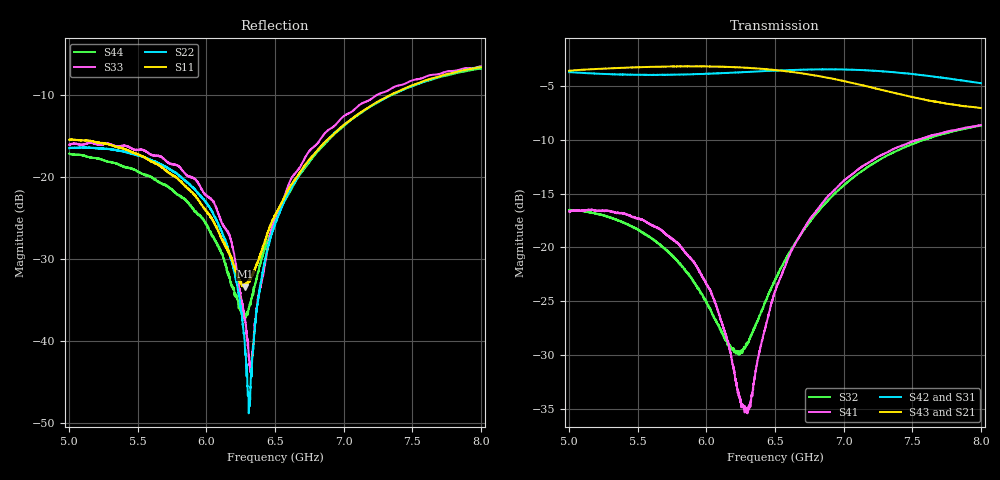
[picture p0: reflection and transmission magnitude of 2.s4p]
!Keysight Technologies,N5225A,MY51451420,A.10.40.12
!Date: Wednesday, May 11, 2016 10:17:49
!Correction: S11(Full 4 Port(1,2,3,4))
!S12(Full 4 Port(1,2,3,4))
!S13(Full 4 Port(1,2,3,4))
!S14(Full 4 Port(1,2,3,4))
!S21(Full 4 Port(1,2,3,4))
!S22(Full 4 Port(1,2,3,4))
!S23(Full 4 Port(1,2,3,4))
!S24(Full 4 Port(1,2,3,4))
!S31(Full 4 Port(1,2,3,4))
!S32(Full 4 Port(1,2,3,4))
!S33(Full 4 Port(1,2,3,4))
!S34(Full 4 Port(1,2,3,4))
!S41(Full 4 Port(1,2,3,4))
!S42(Full 4 Port(1,2,3,4))
!S43(Full 4 Port(1,2,3,4))
!S44(Full 4 Port(1,2,3,4))
!S4P File: Measurements: <S11,S12,S13,S14>,
!<S21,S22,S23,S24>,
!<S31,S32,S33,S34>,
!<S41,S42,S43,S44>:
# Hz S  dB  R 50
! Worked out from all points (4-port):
!   3201 points, 5 GHz to 8 GHz, reference 50 ohm
!   strongest paths, dB at 5 GHz, 5.75 GHz, 6.5 GHz, 7.25 GHz, 8 GHz:
!     S43: -3.6, -3.2, -3.5, -5.3, -7.0
!     S21: -3.6, -3.2, -3.5, -5.2, -7.1
!     S42: -3.7, -3.9, -3.6, -3.6, -4.7
!     S31: -3.8, -4.0, -3.6, -3.7, -4.8
!     S41: -16.7, -19.2, -24.1, -11.6, -8.6
!     S32: -16.5, -20.7, -23.0, -11.9, -8.7
!   lowest |S11| = -33.4 dB at 6.283 GHz (marker M1), VSWR 1.04, Z = 50.8 + j2.02 ohm
!   |S11| at or under -10 dB: start of sweep to 7.336 GHz
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5e9  -15.44 12.8  -3.62 104.7  -3.78 9.8  -16.65 171.5
     -3.62 104.7  -16.47 -113.1  -16.51 -78.1  -3.70 128.3
     -3.77 9.8  -16.50 -78.1  -16.06 -133.0  -3.56 -143.9
     -16.66 171.5  -3.71 128.3  -3.57 -143.9  -17.14 -121.3
5.691875e9  -18.99 -107.9  -3.22 7.5  -4.01 -86.6  -18.60 84.8
            -3.22 7.4  -18.66 162.0  -20.10 -142.1  -3.96 47.9
            -4.01 -86.6  -20.06 -142.0  -17.83 145.0  -3.19 134.1
            -18.61 84.8  -3.95 47.9  -3.19 134.1  -20.94 149.3
6.11e9  -27.42 158.3  -3.22 -52.0  -3.82 -145.9  -26.93 37.7
        -3.23 -52.0  -26.59 106.4  -27.87 -155.0  -3.81 -1.4
        -3.83 -146.0  -27.85 -155.0  -25.53 102.0  -3.21 84.0
        -26.89 37.6  -3.80 -1.5  -3.20 84.0  -29.22 84.7
6.283438e9  -33.37 67.8  -3.32 -76.9  -3.72 -171.1  -34.98 78.4
            -3.32 -76.9  -41.04 55.4  -29.28 -117.3  -3.70 -22.4
            -3.72 -171.1  -29.23 -117.5  -37.56 92.4  -3.29 63.0
            -35.05 77.9  -3.70 -22.4  -3.30 63.0  -36.77 -10.7
6.9875e9  -13.84 -146.8  -4.47 -176.7  -3.53 83.3  -13.96 56.2
          -4.47 -176.7  -13.82 -178.5  -14.38 -143.6  -3.46 -111.2
          -3.54 83.2  -14.39 -143.7  -12.75 175.6  -4.50 -21.3
          -13.96 56.2  -3.46 -111.2  -4.50 -21.3  -13.95 -177.1
7.47875e9  -8.92 126.7  -5.85 118.3  -3.99 8.5  -10.26 -15.7
           -5.85 118.3  -9.00 120.1  -10.52 159.3  -3.86 -174.7
           -3.98 8.6  -10.52 159.4  -8.33 115.0  -5.97 -74.5
           -10.25 -15.7  -3.85 -174.7  -5.96 -74.6  -9.04 116.9
8e9  -6.57 43.9  -7.12 55.1  -4.83 -68.2  -8.63 -87.5
     -7.12 55.1  -6.53 60.4  -8.70 100.1  -4.73 120.2
     -4.82 -68.2  -8.69 100.2  -6.46 51.5  -7.03 -124.8
     -8.62 -87.5  -4.74 120.2  -7.04 -124.8  -6.75 51.8
